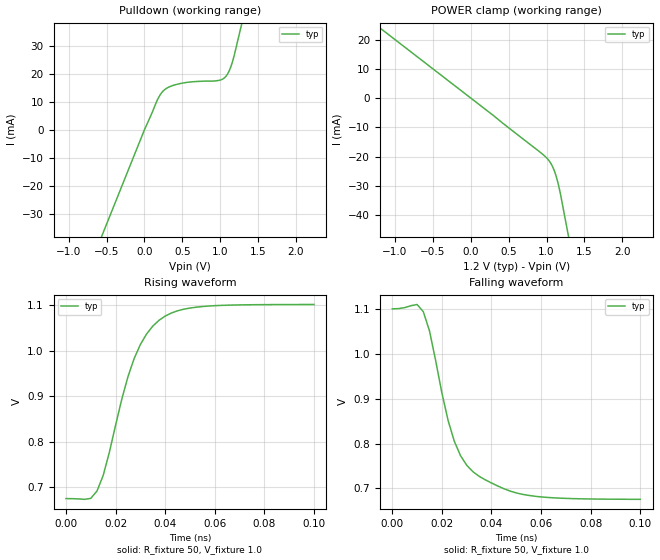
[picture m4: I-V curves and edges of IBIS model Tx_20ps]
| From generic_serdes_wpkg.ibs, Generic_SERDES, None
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[Model]   Tx_20ps
Model_type  Open_sink
C_comp 1.0p  NA  NA
Cref = 0
Vref = 0.8
Rref = 50
Vmeas = 0.8
[Temperature_Range]  25   100   0
[Voltage Range]   1.2   1.14  1.26
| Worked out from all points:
|   slope of the pulldown table from 0 to 0.18 V, typ, clamps not added: 16.1 ohm
|   falling waveform, R_fixture 50, V_fixture 1.0: 20-80 % time 12.6ps typ, NA min, NA max; typ from 1.1 V to 0.675 V
|   rising waveform, R_fixture 50, V_fixture 1.0: 20-80 % time 13.6ps typ, NA min, NA max; typ from 0.675 V to 1.1 V
[Pulldown]
-1.2V     -80.86mA   NA         NA
0V        0A         NA         NA
180mV     11.16mA    NA         NA
270mV     14.38mA    NA         NA
360mV     15.65mA    NA         NA
520mV     16.73mA    NA         NA
1.01V     17.8mA     NA         NA
1.06V     18.63mA    NA         NA
1.11V     20.57mA    NA         NA
1.16V     24.13mA    NA         NA
1.2V      28.29mA    NA         NA
2.4V      165.4mA    NA         NA
[POWER Clamp]
-1.2V     24mA       NA         NA
300mV     -6mA       NA         NA
975mV     -19.81mA   NA         NA
1.05V     -22.08mA   NA         NA
1.1V      -24.74mA   NA         NA
1.13V     -27.08mA   NA         NA
1.15V     -29mA      NA         NA
1.17V     -31.22mA   NA         NA
1.2V      -35.12mA   NA         NA
2.4V      -199.3mA   NA         NA
[Ramp]
| variable   typ   min   max
dV/dt_r   0.256/1.3595E-11   NA   NA
dV/dt_f   0.256/1.2625E-11   NA   NA
R_load = 50ohms
[Falling Waveform]
R_fixture = 50
V_fixture = 1.0
| Time   V(typ)   V(min)  V(max)
0s        1.101V     NA         NA
10ps      1.111V     NA         NA
12.5ps    1.095V     NA         NA
15ps      1.052V     NA         NA
20ps      913.1mV    NA         NA
25ps      805.2mV    NA         NA
27.5ps    773mV      NA         NA
32.5ps    737mV      NA         NA
55ps      683.9mV    NA         NA
100ps     675.1mV    NA         NA
[Rising Waveform]
R_fixture = 50
V_fixture = 1.0
| Time   V(typ)   V(min)  V(max)
0s        674.9mV    NA         NA
10ps      675.4mV    NA         NA
12.5ps    691.3mV    NA         NA
15ps      725.4mV    NA         NA
22.5ps    892.7mV    NA         NA
27.5ps    982.3mV    NA         NA
32.5ps    1.036V     NA         NA
37.5ps    1.066V     NA         NA
55ps      1.097V     NA         NA
100ps     1.101V     NA         NA
[Algorithmic Model]
Executable   Windows_VisualStudio_32   MentorTx_32.dll   MentorTx.ami
Executable   Windows_VisualStudio_64   MentorTx_64.dll   MentorTx.ami
Executable   Linux_gcc3.2.3_32   libMentorTx_32.so   MentorTx.ami
Executable   Linux_gcc3.2.3_64   libMentorTx_64.so   MentorTx.ami
[End Algorithmic Model]
